ORGANIZATION_BLOCK "CycleExecution"
TITLE =
VERSION : 0.1


VAR_TEMP
  OB1_EV_CLASS : BYTE ;	//Bits 0-3 = 1 (Coming event), Bits 4-7 = 1 (Event class 1)
  OB1_SCAN_1 : BYTE ;	//1 (Cold restart scan 1 of OB 1), 3 (Scan 2-n of OB 1)
  OB1_PRIORITY : BYTE ;	//1 (Priority of 1 is lowest)
  OB1_OB_NUMBR : BYTE ;	//1 (Organization block 1, OB1)
  OB1_RESERVED_1 : BYTE ;	//Reserved for system
  OB1_RESERVED_2 : BYTE ;	//Reserved for system
  OB1_PREV_CYCLE : INT ;	//Cycle time of previous OB1 scan (milliseconds)
  OB1_MIN_CYCLE : INT ;	//Minimum cycle time of OB1 (milliseconds)
  OB1_MAX_CYCLE : INT ;	//Maximum cycle time of OB1 (milliseconds)
  OB1_DATE_TIME : DATE_AND_TIME ;	//Date and time OB1 started
END_VAR
BEGIN
NETWORK
TITLE =Chiamata condizioni generali

      CALL "GeneralConditions" ;
      NOP   0;
NETWORK
TITLE =Chiamata funzioni caricatore

      CALL "FC-callsLoader" ;
      NOP   0;
NETWORK
TITLE =Chiamata funzioni pressa

      CALL "FC-callsPress" ;
      NOP   0;
NETWORK
TITLE =Chiamata funzione destacker

      CALL "Interface Destacker" ;
      NOP   0;
NETWORK
TITLE =Chiamata funzioni robot

      CALL "Interface Robot" ;
      NOP   0;
NETWORK
TITLE =chiamata funzioni programma principale

      CALL "ProgramManagement" ;
      NOP   0;
END_ORGANIZATION_BLOCK

